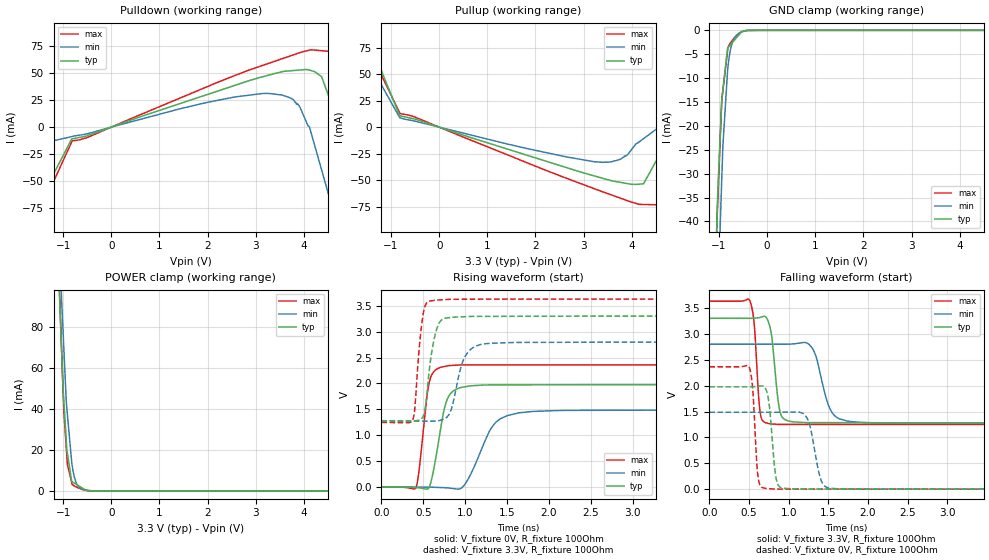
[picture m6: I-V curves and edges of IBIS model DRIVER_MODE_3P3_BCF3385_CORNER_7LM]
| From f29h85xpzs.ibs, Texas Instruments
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|   Model Cell DRIVER_MODE_3P3_BCF3385_CORNER_7LM
|DRIVER_MODE_3P3_BCF3385_CORNER_7LM
[Model]   DRIVER_MODE_3P3_BCF3385_CORNER_7LM
Model_type   I/O
Polarity   Non-Inverting
Enable   Active-Low
Vinl = 0.8
Vinh = 2
Vmeas = 1.65
Vref = 0
Cref = 15pF
Rref = 100M
|   typ   min   max
C_comp   0.44pF   0.4pF   0.46pF
[Model Spec]
Vinl   0.8   0.8   0.8
Vinh   2   2   2
[Temperature Range]   25   155   -40
[Voltage Range]   3.3   2.8   3.63
| Nom Voltages:
|   BIASFET=3.3, VDD=1.23, VDDS=3.3, VSS=0
| Min Voltages:
|   BIASFET=2.97, VDD=1.08, VDDS=2.8, VSS=0
| Max Voltages:
|   BIASFET=3.63, VDD=1.32, VDDS=3.63, VSS=0
[Pullup Reference]   3.3   2.8   3.63
[Pulldown Reference]   0   0   0
[Power Clamp Reference]   3.3   2.8   3.63
[GND Clamp Reference]   0   0   0
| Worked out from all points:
|   slope of the pulldown table from 0 to 0.495 V, typ, clamps not added: 62.6 ohm
|   slope of the pullup table from 0 to 0.495 V, typ, clamps not added: 66 ohm
|   GND clamp passes 1 mA (typ) near -0.59 V on its own axis
|   POWER clamp passes 1 mA (typ) near -0.57 V on its own axis
|   falling waveform, V_fixture 3.3V, R_fixture 100Ohm: 20-80 % time 78.5ps typ, 156ps min, 56.9ps max; typ from 3.3 V to 1.28 V
|   rising waveform, V_fixture 0V, R_fixture 100Ohm: 20-80 % time 132ps typ, 253ps min, 96ps max; typ from 0 V to 1.98 V
|   rising waveform, V_fixture 3.3V, R_fixture 100Ohm: 20-80 % time 99.7ps typ, 143ps min, 73.2ps max; typ from 1.28 V to 3.3 V
|   falling waveform, V_fixture 0V, R_fixture 100Ohm: 20-80 % time 66ps typ, 111ps min, 51ps max; typ from 1.98 V to 0 V
[Pulldown]
|   Voltage   I(typ)   I(min)   I(max)
-3.3V     -6.486mA   -1.715mA   -9.548mA
-3.215V   -57.46mA   -41.28mA   -93.25mA
-2.155V   -75.14mA   -54.81mA   -103.1mA
-813.2mV  -10.83mA   -8.657mA   -12.73mA
3.548V    51.23mA    29.71mA    63.28mA
4.602V    18.03mA    -76.16mA   66.74mA
6.076V    -45.99mA   -97.61mA   -23.27mA
6.172V    -46.75mA   -22.33mA   -29.14mA
6.504V    -49.38mA   -121.2mA   -49.38mA
6.508V    -49.42mA   -122.1mA   41.27mA
6.521V    -49.52mA   290mA      288.5mA
6.6V      1.963A     2.877A     1.84A
[GND Clamp]
|   Voltage   I(typ)   I(min)   I(max)
-3.3V     -1.475A    -1.211A    -2.162A
-1.049V   -43.36mA   -65.77mA   -41.74mA
-1.034V   -36.84mA   -59.68mA   -37.95mA
-1.021V   -32.89mA   -54.96mA   -34.73mA
-942.1mV  -14.63mA   -31.04mA   -14.52mA
-919.6mV  -12.6mA    -24.26mA   -12.61mA
-821.6mV  -3.732mA   -8.468mA   -4.288mA
-813.2mV  -3.634mA   -7.599mA   -3.582mA
-760.2mV  -3.01mA    -4.001mA   -2.612mA
-695.6mV  -2.251mA   -1.907mA   -1.765mA
-520.2mV  -187uA     -304.1uA   -267uA
6.6V      0A         0A         0A
[Pullup]
|   Voltage   I(typ)   I(min)   I(max)
-3.3V     6.741mA    2.485mA    9.999mA
-3.13V    87.18mA    89.61mA    102.7mA
-2.155V   94.97mA    100.2mA    99.18mA
-1.561V   93.69mA    98.59mA    79.29mA
-1.383V   73.68mA    22.13mA    66.35mA
-821.6mV  10.72mA    9.079mA    13.54mA
3.234V    -46.23mA   -32.8mA    -58.36mA
4.604V    -23.84mA   1.255mA    -73.46mA
6.504V    21.4mA     65.24mA    35.68mA
6.508V    21.42mA    66mA       -56.95mA
6.521V    21.49mA    -156.8mA   -309.5mA
6.6V      -1.505A    -1.555A    -1.895A
[POWER Clamp]
|   Voltage   I(typ)   I(min)   I(max)
-3.3V     1.946A     2.25A      2.109A
-1.089V   103.2mA    134.1mA    106.2mA
-1.042V   74.06mA    99.42mA    74.93mA
-1.031V   67.61mA    92.78mA    68.01mA
-1.008V   53.33mA    80.96mA    52.68mA
-985.9mV  43.87mA    69.53mA    38.7mA
-933.8mV  24.02mA    42.92mA    20.37mA
-912.5mV  18.3mA     37.4mA     12.88mA
-821.6mV  4.553mA    13.81mA    4.028mA
-800.3mV  4.248mA    10.51mA    2.95mA
-658.3mV  2.214mA    1.599mA    1.195mA
6.6V      0A         0A         0A
[Ramp]
R_load = 100
|   typ   min   max
dV/dt_r   1.18626/1.31596e-10   0.891141/2.52422e-10   1.41848/9.59061e-11
dV/dt_f   1.21095/7.85471e-11   0.91513/1.555e-10   1.42951/5.68546e-11
[Falling Waveform]
V_fixture = 3.3V
V_fixture_min = 2.8V
V_fixture_max = 3.63V
R_fixture = 100Ohm
C_fixture = 0F
|   Time   V(typ)   V(min)   V(max)
0s        3.3V       2.8V       3.63V
506.2ps   3.3V       2.8V       3.651V
563.4ps   3.3V       2.8V       3.228V
652.1ps   3.324V     2.8V       1.39V
773.8ps   3.065V     2.8V       1.261V
857.7ps   1.827V     2.8V       1.251V
1.258ns   1.286V     2.795V     1.251V
1.572ns   1.285V     1.431V     1.251V
2.056ns   1.283V     1.282V     1.251V
50ns      1.282V     1.275V     1.247V
[Rising Waveform]
V_fixture = 0V
V_fixture_min = 0V
V_fixture_max = 0V
R_fixture = 100Ohm
C_fixture = 0F
|   Time   V(typ)   V(min)   V(max)
0s        1.941uV    2.93uV     8.714nV
414.3ps   -9.953mV   -1.356mV   -3.398mV
447.8ps   -13.54mV   -1.466mV   304.6mV
563.7ps   -22.05mV   -1.846mV   1.962V
619.9ps   305.3mV    -3.068mV   2.218V
773.8ps   1.643V     -14.11mV   2.335V
957.4ps   1.925V     -14.82mV   2.36V
1.398ns   1.973V     1.293V     2.36V
2.133ns   1.975V     1.479V     2.36V
50ns      1.977V     1.485V     2.364V
[Rising Waveform]
V_fixture = 3.3V
V_fixture_min = 2.8V
V_fixture_max = 3.63V
R_fixture = 100Ohm
C_fixture = 0F
|   Time   V(typ)   V(min)   V(max)
0s        1.282V     1.275V     1.247V
373.4ps   1.28V      1.273V     1.297V
399.5ps   1.28V      1.272V     1.538V
487.4ps   1.335V     1.272V     3.224V
536.9ps   1.71V      1.272V     3.548V
650ps     2.999V     1.277V     3.609V
807.7ps   3.27V      1.403V     3.624V
1.048ns   3.293V     2.632V     3.627V
1.615ns   3.297V     2.792V     3.63V
50ns      3.3V       2.8V       3.63V
[Falling Waveform]
|Gnd
V_fixture = 0V
V_fixture_min = 0V
V_fixture_max = 0V
R_fixture = 100Ohm
C_fixture = 0F
|   Time   V(typ)   V(min)   V(max)
0s        1.977V     1.485V     2.364V
498.6ps   1.977V     1.485V     2.37V
619.9ps   1.988V     1.485V     180.3mV
739.5ps   1.788V     1.485V     10.97mV
807.7ps   672.3mV    1.485V     3.314mV
883.9ps   46.32mV    1.486V     2.075mV
1.21ns    3.804mV    1.424V     176.2uV
1.428ns   3.308mV    110.8mV    3.205uV
1.696ns   2.698mV    5.15mV     3.187uV
50ns      1.941uV    2.93uV     32.99nV
